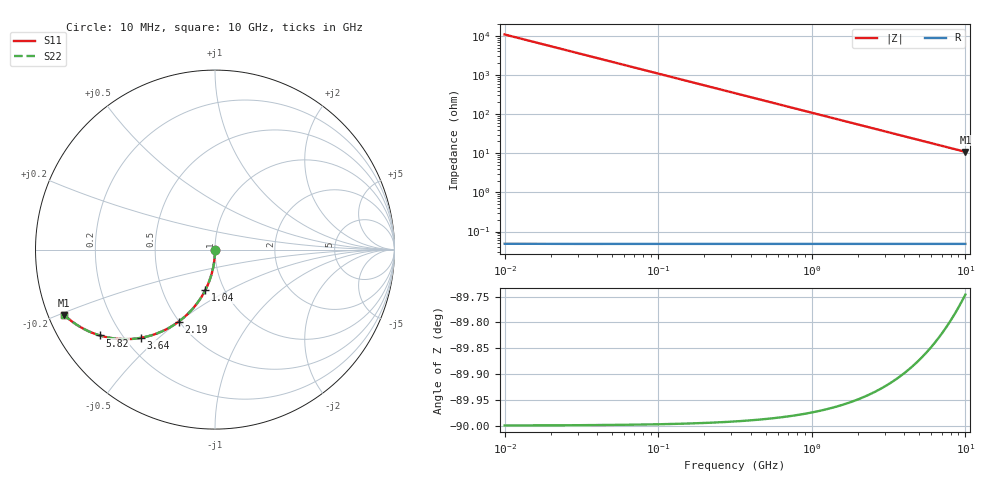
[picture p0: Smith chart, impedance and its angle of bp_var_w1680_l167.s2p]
! Created Wed Nov  4 11:47:11 2020
# ghz S ma R 50
! 2 Port Network Data from SP1.SP block
! freq  magS11  angS11  magS21  angS21  magS12  angS12  magS22  angS22
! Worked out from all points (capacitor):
!   1000 points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, 10 MHz to 10 GHz, reference 50 ohm
!   read as one part in shunt: C = 1.46 pF near 60 MHz
!   lowest |Z| = 10.9 ohm at 10 GHz (marker M1)
!   S11 on the Smith chart (normalised r, x): 10 MHz: 1.00, -0.00; 1.04 GHz: 0.81, -0.39; 2.19 GHz: 0.50, -0.50; 3.64 GHz: 0.26, -0.44; 5.82 GHz: 0.12, -0.33; 10 GHz: 0.05, -0.21
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0.01  0.002299 -90.1  1 -0.1  1 -0.1  0.002299 -90.1
0.04  0.009195 -90.5  1 -0.5  1 -0.5  0.009195 -90.5
0.07  0.01609 -90.9  0.9999 -0.9  0.9999 -0.9  0.01609 -90.9
0.08  0.01839 -91.1  0.9998 -1.1  0.9998 -1.1  0.01839 -91.1
0.1  0.02298 -91.3  0.9997 -1.3  0.9997 -1.3  0.02298 -91.3
0.13  0.02987 -91.7  0.9996 -1.7  0.9996 -1.7  0.02987 -91.7
0.17  0.03905 -92.2  0.9992 -2.2  0.9992 -2.2  0.03905 -92.2
0.26  0.05967 -93.4  0.9982 -3.4  0.9982 -3.4  0.05967 -93.4
0.39  0.0893 -95.1  0.996 -5.1  0.996 -5.1  0.0893 -95.1
0.56  0.1277 -97.3  0.9918 -7.3  0.9918 -7.3  0.1277 -97.3
0.78  0.1765 -100.2  0.9842 -10.2  0.9842 -10.2  0.1765 -100.2
1.04  0.2325 -103.5  0.9725 -13.4  0.9725 -13.4  0.2325 -103.5
1.34  0.2944 -107.2  0.9555 -17.1  0.9555 -17.1  0.2944 -107.2
1.68  0.3602 -111.2  0.9326 -21.1  0.9326 -21.1  0.3602 -111.2
2.19  0.4495 -116.8  0.8928 -26.7  0.8928 -26.7  0.4495 -116.8
3.34  0.6086 -127.6  0.7926 -37.5  0.7926 -37.5  0.6086 -127.6
3.64  0.6413 -130.0  0.7663 -39.9  0.7663 -39.9  0.6413 -130.0
5.01  0.7543 -139.1  0.6549 -49.0  0.6549 -49.0  0.7543 -139.1
5.82  0.8 -143.3  0.5979 -53.1  0.5979 -53.1  0.8 -143.3
6.67  0.8365 -146.9  0.5455 -56.8  0.5455 -56.8  0.8365 -146.9
8.34  0.8853 -152.5  0.4617 -62.3  0.4617 -62.3  0.8853 -152.5
10  0.9155 -156.5  0.3982 -66.3  0.3982 -66.3  0.9155 -156.5
